FUNCTION "Gest Aut Boxing SX" : VOID
TITLE =Gestione Automatico Boxing SX
AUTHOR : MassimoZ
FAMILY : NovaSrl
VERSION : 0.1

BEGIN
NETWORK
TITLE ======== Automatico Pintaggio Elementi Boxing SX ======



NETWORK
TITLE =Presenza Pezzo su Dosatore in Entrata Boxing SX

      U(    ;
      UN    "SL710";
      U     "SL710B";
      U     "FT502";
      L     S5T#500MS;
      SE    T     86;
      NOP   0;
      NOP   0;
      NOP   0;
      U     T     86;
      )     ;
      L     S5T#700MS;
      SA    T     87;
      NOP   0;
      NOP   0;
      NOP   0;
      U     T     87;
      =     "M90.0";
NETWORK
TITLE =Presenza Pezzo su Prima Zona di Lavoro Boxing SX

      U(    ;
      UN    "SL710";
      U     "SL710B";
      U     "FT504";
      L     S5T#500MS;
      SE    T     88;
      NOP   0;
      NOP   0;
      NOP   0;
      U     T     88;
      )     ;
      L     S5T#300MS;
      SA    T     89;
      NOP   0;
      NOP   0;
      NOP   0;
      U     T     89;
      =     "M90.1";
NETWORK
TITLE =Presenza Pezzo su Seconda Zona di Lavoro Boxing SX

      U(    ;
      UN    "SL710";
      U     "SL710B";
      U     "FT506";
      L     S5T#500MS;
      SE    T     90;
      NOP   0;
      NOP   0;
      NOP   0;
      U     T     90;
      )     ;
      L     S5T#300MS;
      SA    T     91;
      NOP   0;
      NOP   0;
      NOP   0;
      U     T     91;
      =     "M90.2";
NETWORK
TITLE =Presenza Pezzo su Terza Zona di Lavoro Boxing SX

      U(    ;
      UN    "SL710";
      U     "SL710B";
      U     "FT510";
      L     S5T#500MS;
      SE    T     92;
      NOP   0;
      NOP   0;
      NOP   0;
      U     T     92;
      )     ;
      L     S5T#300MS;
      SA    T     93;
      NOP   0;
      NOP   0;
      NOP   0;
      U     T     93;
      =     "M90.3";
NETWORK
TITLE =Com Aut Start Motore Nastro 3
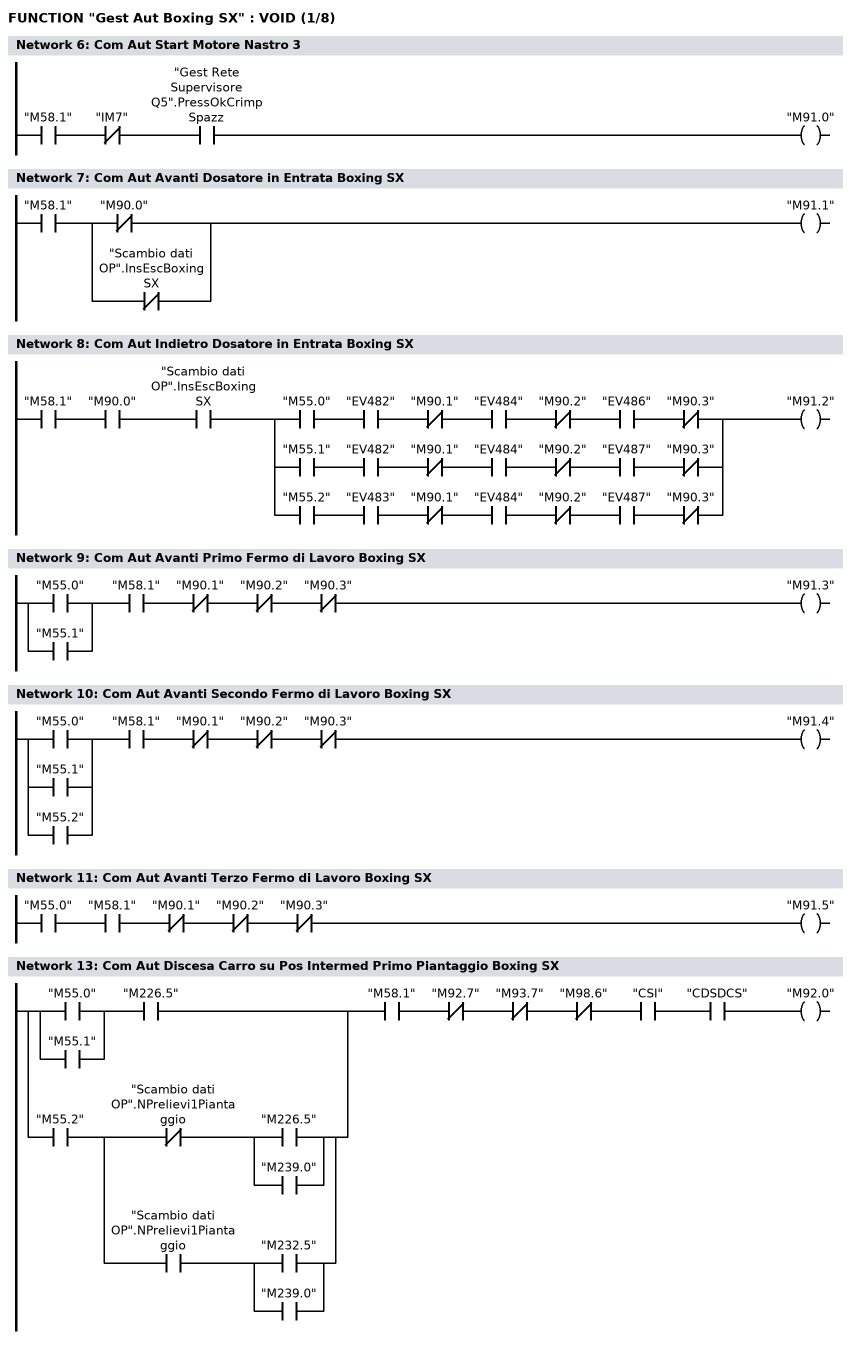
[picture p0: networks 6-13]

      U     "M58.1";
      UN    "IM7";
      U     "Gest Rete Supervisore Q5".PressOkCrimpSpazz;
      =     "M91.0";
NETWORK
TITLE =Com Aut Avanti Dosatore in Entrata Boxing SX

      U     "M58.1";
      U(    ;
      ON    "M90.0";
      ON    "Scambio dati OP".InsEscBoxingSX;
      )     ;
      =     "M91.1";
NETWORK
TITLE =Com Aut Indietro Dosatore in Entrata Boxing SX

      U     "M58.1";
      U     "M90.0";
      U     "Scambio dati OP".InsEscBoxingSX;
      U(    ;
      U     "M55.0";
      U     "EV482";
      UN    "M90.1";
      U     "EV484";
      UN    "M90.2";
      U     "EV486";
      UN    "M90.3";
      O     ;
      U     "M55.1";
      U     "EV482";
      UN    "M90.1";
      U     "EV484";
      UN    "M90.2";
      U     "EV487";
      UN    "M90.3";
      O     ;
      U     "M55.2";
      U     "EV483";
      UN    "M90.1";
      U     "EV484";
      UN    "M90.2";
      U     "EV487";
      UN    "M90.3";
      )     ;
      =     "M91.2";
NETWORK
TITLE =Com Aut Avanti Primo Fermo di Lavoro Boxing SX

      U(    ;
      O     "M55.0";
      O     "M55.1";
      )     ;
      U     "M58.1";
      UN    "M90.1";
      UN    "M90.2";
      UN    "M90.3";
      =     "M91.3";
NETWORK
TITLE =Com Aut Avanti Secondo Fermo di Lavoro Boxing SX

      U(    ;
      O     "M55.0";
      O     "M55.1";
      O     "M55.2";
      )     ;
      U     "M58.1";
      UN    "M90.1";
      UN    "M90.2";
      UN    "M90.3";
      =     "M91.4";
NETWORK
TITLE =Com Aut Avanti Terzo Fermo di Lavoro Boxing SX

      U     "M55.0";
      U     "M58.1";
      UN    "M90.1";
      UN    "M90.2";
      UN    "M90.3";
      =     "M91.5";
NETWORK
TITLE ======= Primo Piantag per Batterie 12V 16V e Batterie in Linea ==



NETWORK
TITLE =Com Aut Discesa Carro su Pos Intermed Primo Piantaggio Boxing SX

      U(    ;
      U(    ;
      O     "M55.0";
      O     "M55.1";
      )     ;
      U     "M226.5";
      O     ;
      U     "M55.2";
      U(    ;
      UN    "Scambio dati OP".NPrelievi1Piantaggio;
      U(    ;
      O     "M226.5";
      O     "M239.0";
      )     ;
      O     ;
      U     "Scambio dati OP".NPrelievi1Piantaggio;
      U(    ;
      O     "M232.5";
      O     "M239.0";
      )     ;
      )     ;
      )     ;
      U     "M58.1";
      UN    "M92.7";
      UN    "M93.7";
      UN    "M98.6";
      U     "CSI";
      U     "CDSDCS";
      =     "M92.0";
NETWORK
TITLE =Com Aut Avanti Carro Primo Piantaggio Boxing SX
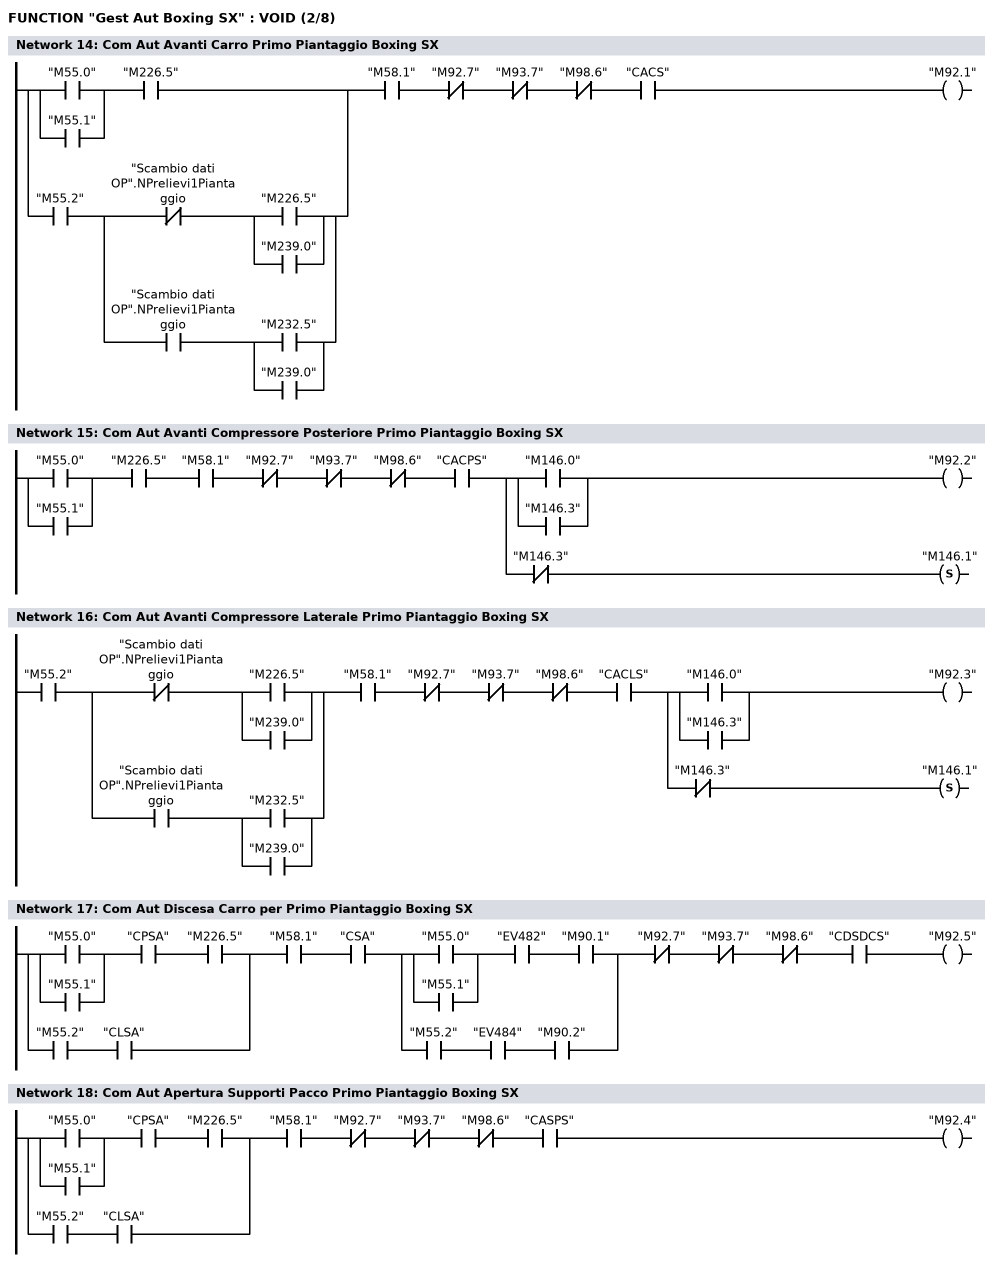
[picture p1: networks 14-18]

      U(    ;
      U(    ;
      O     "M55.0";
      O     "M55.1";
      )     ;
      U     "M226.5";
      O     ;
      U     "M55.2";
      U(    ;
      UN    "Scambio dati OP".NPrelievi1Piantaggio;
      U(    ;
      O     "M226.5";
      O     "M239.0";
      )     ;
      O     ;
      U     "Scambio dati OP".NPrelievi1Piantaggio;
      U(    ;
      O     "M232.5";
      O     "M239.0";
      )     ;
      )     ;
      )     ;
      U     "M58.1";
      UN    "M92.7";
      UN    "M93.7";
      UN    "M98.6";
      U     "CACS";
      =     "M92.1";
NETWORK
TITLE =Com Aut Avanti Compressore Posteriore Primo Piantaggio Boxing SX

      U(    ;
      O     "M55.0";
      O     "M55.1";
      )     ;
      U     "M226.5";
      U     "M58.1";
      UN    "M92.7";
      UN    "M93.7";
      UN    "M98.6";
      U     "CACPS";
      =     L      0.0;
      U     L      0.0;
      U(    ;
      O     "M146.0";
      O     "M146.3";
      )     ;
      =     "M92.2";
      U     L      0.0;
      UN    "M146.3";
      S     "M146.1";
NETWORK
TITLE =Com Aut Avanti Compressore Laterale Primo Piantaggio Boxing SX

      U     "M55.2";
      U(    ;
      UN    "Scambio dati OP".NPrelievi1Piantaggio;
      U(    ;
      O     "M226.5";
      O     "M239.0";
      )     ;
      O     ;
      U     "Scambio dati OP".NPrelievi1Piantaggio;
      U(    ;
      O     "M232.5";
      O     "M239.0";
      )     ;
      )     ;
      U     "M58.1";
      UN    "M92.7";
      UN    "M93.7";
      UN    "M98.6";
      U     "CACLS";
      =     L      0.0;
      U     L      0.0;
      U(    ;
      O     "M146.0";
      O     "M146.3";
      )     ;
      =     "M92.3";
      U     L      0.0;
      UN    "M146.3";
      S     "M146.1";
NETWORK
TITLE =Com Aut Discesa Carro per Primo Piantaggio Boxing SX

      U(    ;
      U(    ;
      O     "M55.0";
      O     "M55.1";
      )     ;
      U     "CPSA";
      U     "M226.5";
      O     ;
      U     "M55.2";
      U     "CLSA";
      )     ;
      U     "M58.1";
      U     "CSA";
      U(    ;
      U(    ;
      O     "M55.0";
      O     "M55.1";
      )     ;
      U     "EV482";
      U     "M90.1";
      O     ;
      U     "M55.2";
      U     "EV484";
      U     "M90.2";
      )     ;
      UN    "M92.7";
      UN    "M93.7";
      UN    "M98.6";
      U     "CDSDCS";
      =     "M92.5";
NETWORK
TITLE =Com Aut Apertura Supporti Pacco Primo Piantaggio Boxing SX

      U(    ;
      U(    ;
      O     "M55.0";
      O     "M55.1";
      )     ;
      U     "CPSA";
      U     "M226.5";
      O     ;
      U     "M55.2";
      U     "CLSA";
      )     ;
      U     "M58.1";
      UN    "M92.7";
      UN    "M93.7";
      UN    "M98.6";
      U     "CASPS";
      =     "M92.4";
NETWORK
TITLE =Com Aut Avanti Blocc Pezzo Zona Lavoro Primo Piantagg Boxing SX
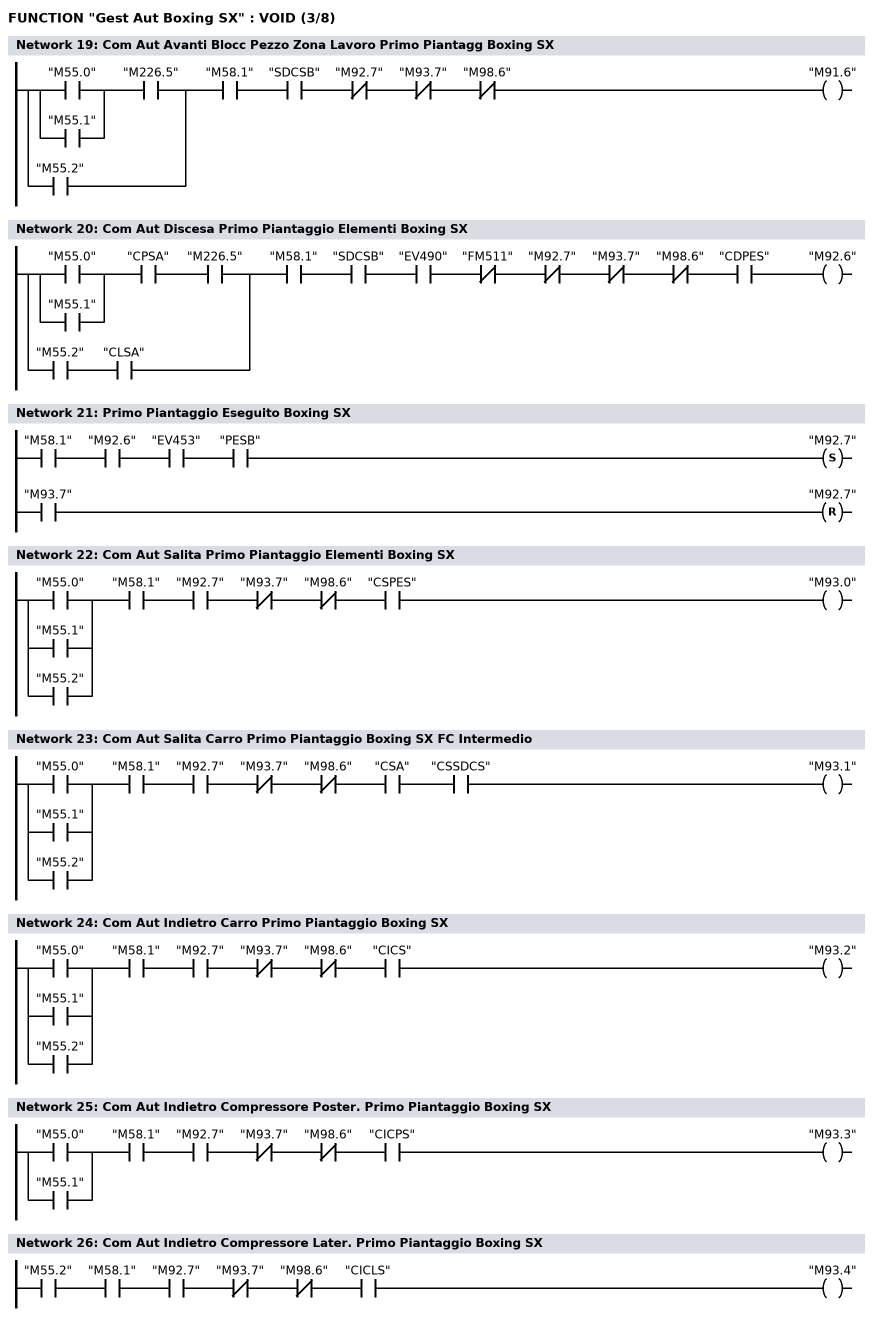
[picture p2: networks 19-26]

      U(    ;
      U(    ;
      O     "M55.0";
      O     "M55.1";
      )     ;
      U     "M226.5";
      O     "M55.2";
      )     ;
      U     "M58.1";
      U     "SDCSB";
      UN    "M92.7";
      UN    "M93.7";
      UN    "M98.6";
      =     "M91.6";
NETWORK
TITLE =Com Aut Discesa Primo Piantaggio Elementi Boxing SX

      U(    ;
      U(    ;
      O     "M55.0";
      O     "M55.1";
      )     ;
      U     "CPSA";
      U     "M226.5";
      O     ;
      U     "M55.2";
      U     "CLSA";
      )     ;
      U     "M58.1";
      U     "SDCSB";
      U     "EV490";
      UN    "FM511";
      UN    "M92.7";
      UN    "M93.7";
      UN    "M98.6";
      U     "CDPES";
      =     "M92.6";
NETWORK
TITLE =Primo Piantaggio Eseguito Boxing SX

      U     "M58.1";
      U     "M92.6";
      U     "EV453";
      U     "PESB";
      S     "M92.7";
      U     "M93.7";
      R     "M92.7";
      NOP   0;
NETWORK
TITLE =Com Aut Salita Primo Piantaggio Elementi Boxing SX

      U(    ;
      O     "M55.0";
      O     "M55.1";
      O     "M55.2";
      )     ;
      U     "M58.1";
      U     "M92.7";
      UN    "M93.7";
      UN    "M98.6";
      U     "CSPES";
      =     "M93.0";
NETWORK
TITLE =Com Aut Salita Carro Primo Piantaggio Boxing SX FC Intermedio

      U(    ;
      O     "M55.0";
      O     "M55.1";
      O     "M55.2";
      )     ;
      U     "M58.1";
      U     "M92.7";
      UN    "M93.7";
      UN    "M98.6";
      U     "CSA";
      U     "CSSDCS";
      =     "M93.1";
NETWORK
TITLE =Com Aut Indietro Carro Primo Piantaggio Boxing SX

      U(    ;
      O     "M55.0";
      O     "M55.1";
      O     "M55.2";
      )     ;
      U     "M58.1";
      U     "M92.7";
      UN    "M93.7";
      UN    "M98.6";
      U     "CICS";
      =     "M93.2";
NETWORK
TITLE =Com Aut Indietro Compressore Poster. Primo Piantaggio Boxing SX

      U(    ;
      O     "M55.0";
      O     "M55.1";
      )     ;
      U     "M58.1";
      U     "M92.7";
      UN    "M93.7";
      UN    "M98.6";
      U     "CICPS";
      =     "M93.3";
NETWORK
TITLE =Com Aut Indietro Compressore Later. Primo Piantaggio Boxing SX

      U     "M55.2";
      U     "M58.1";
      U     "M92.7";
      UN    "M93.7";
      UN    "M98.6";
      U     "CICLS";
      =     "M93.4";
NETWORK
TITLE =Com Aut Chiusura Supporto Pacchi Primo Piantaggio Boxing SX
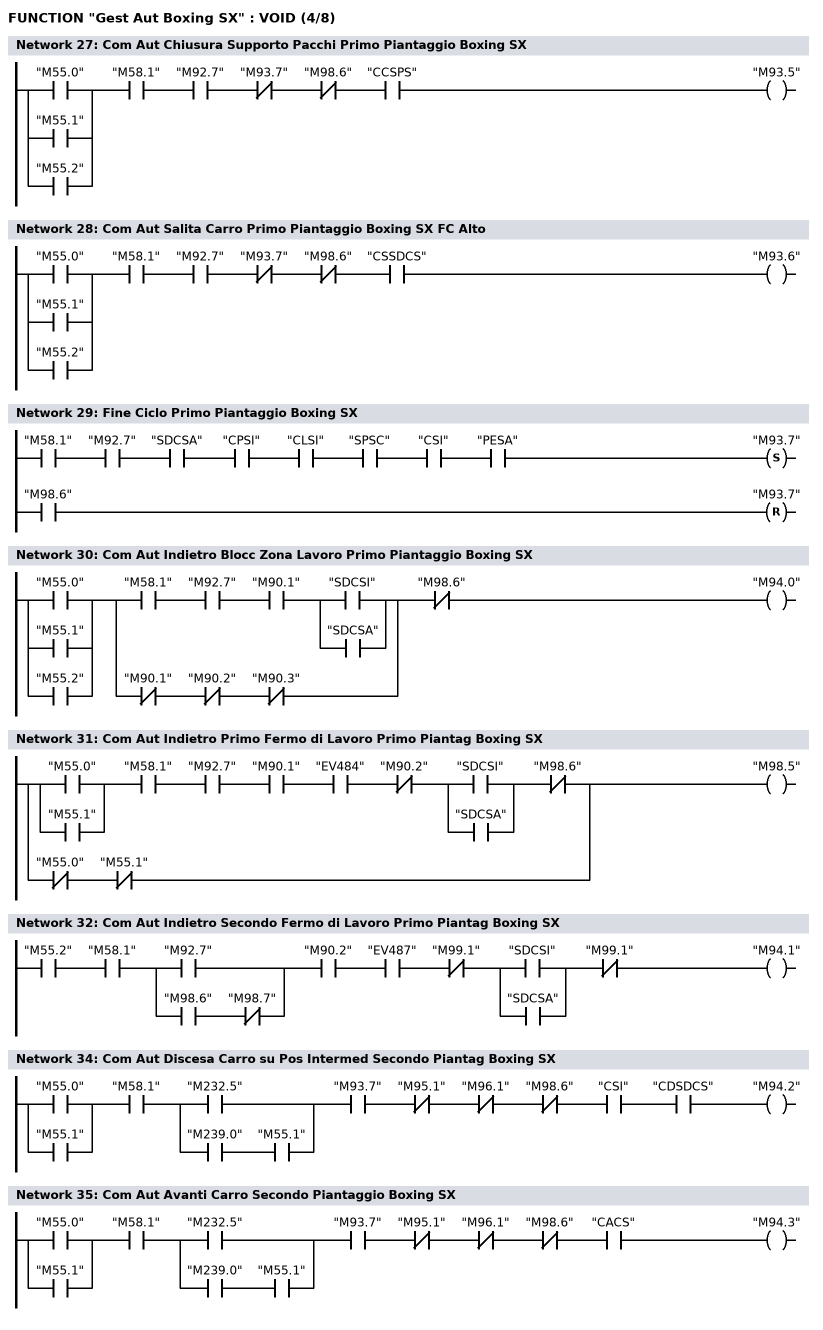
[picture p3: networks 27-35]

      U(    ;
      O     "M55.0";
      O     "M55.1";
      O     "M55.2";
      )     ;
      U     "M58.1";
      U     "M92.7";
      UN    "M93.7";
      UN    "M98.6";
      U     "CCSPS";
      =     "M93.5";
NETWORK
TITLE =Com Aut Salita Carro Primo Piantaggio Boxing SX FC Alto

      U(    ;
      O     "M55.0";
      O     "M55.1";
      O     "M55.2";
      )     ;
      U     "M58.1";
      U     "M92.7";
      UN    "M93.7";
      UN    "M98.6";
      U     "CSSDCS";
      =     "M93.6";
NETWORK
TITLE =Fine Ciclo Primo Piantaggio Boxing SX

      U     "M58.1";
      U     "M92.7";
      U     "SDCSA";
      U     "CPSI";
      U     "CLSI";
      U     "SPSC";
      U     "CSI";
      U     "PESA";
      S     "M93.7";
      U     "M98.6";
      R     "M93.7";
      NOP   0;
NETWORK
TITLE =Com Aut Indietro Blocc Zona Lavoro Primo Piantaggio Boxing SX

      U(    ;
      O     "M55.0";
      O     "M55.1";
      O     "M55.2";
      )     ;
      U(    ;
      U     "M58.1";
      U     "M92.7";
      U     "M90.1";
      U(    ;
      O     "SDCSI";
      O     "SDCSA";
      )     ;
      O     ;
      UN    "M90.1";
      UN    "M90.2";
      UN    "M90.3";
      )     ;
      UN    "M98.6";
      =     "M94.0";
NETWORK
TITLE =Com Aut Indietro Primo Fermo di Lavoro Primo Piantag Boxing SX

      U(    ;
      O     "M55.0";
      O     "M55.1";
      )     ;
      U     "M58.1";
      U     "M92.7";
      U     "M90.1";
      U     "EV484";
      UN    "M90.2";
      U(    ;
      O     "SDCSI";
      O     "SDCSA";
      )     ;
      UN    "M98.6";
      O     ;
      UN    "M55.0";
      UN    "M55.1";
      =     "M98.5";
NETWORK
TITLE =Com Aut Indietro Secondo Fermo di Lavoro Primo Piantag Boxing SX

      U     "M55.2";
      U     "M58.1";
      U(    ;
      O     "M92.7";
      O     ;
      U     "M98.6";
      UN    "M98.7";
      )     ;
      U     "M90.2";
      U     "EV487";
      UN    "M99.1";
      U(    ;
      O     "SDCSI";
      O     "SDCSA";
      )     ;
      UN    "M99.1";
      =     "M94.1";
NETWORK
TITLE ======= Secondo Pinataggio per Batterie 12V 16V =======



NETWORK
TITLE =Com Aut Discesa Carro su Pos Intermed Secondo Piantag Boxing SX

      U(    ;
      O     "M55.0";
      O     "M55.1";
      )     ;
      U     "M58.1";
      U(    ;
      O     "M232.5";
      O     ;
      U     "M239.0";
      U     "M55.1";
      )     ;
      U     "M93.7";
      UN    "M95.1";
      UN    "M96.1";
      UN    "M98.6";
      U     "CSI";
      U     "CDSDCS";
      =     "M94.2";
NETWORK
TITLE =Com Aut Avanti Carro Secondo Piantaggio Boxing SX

      U(    ;
      O     "M55.0";
      O     "M55.1";
      )     ;
      U     "M58.1";
      U(    ;
      O     "M232.5";
      O     ;
      U     "M239.0";
      U     "M55.1";
      )     ;
      U     "M93.7";
      UN    "M95.1";
      UN    "M96.1";
      UN    "M98.6";
      U     "CACS";
      =     "M94.3";
NETWORK
TITLE =Com Aut Avanti Compressore Posteriore Secondo Piantag Boxing SX
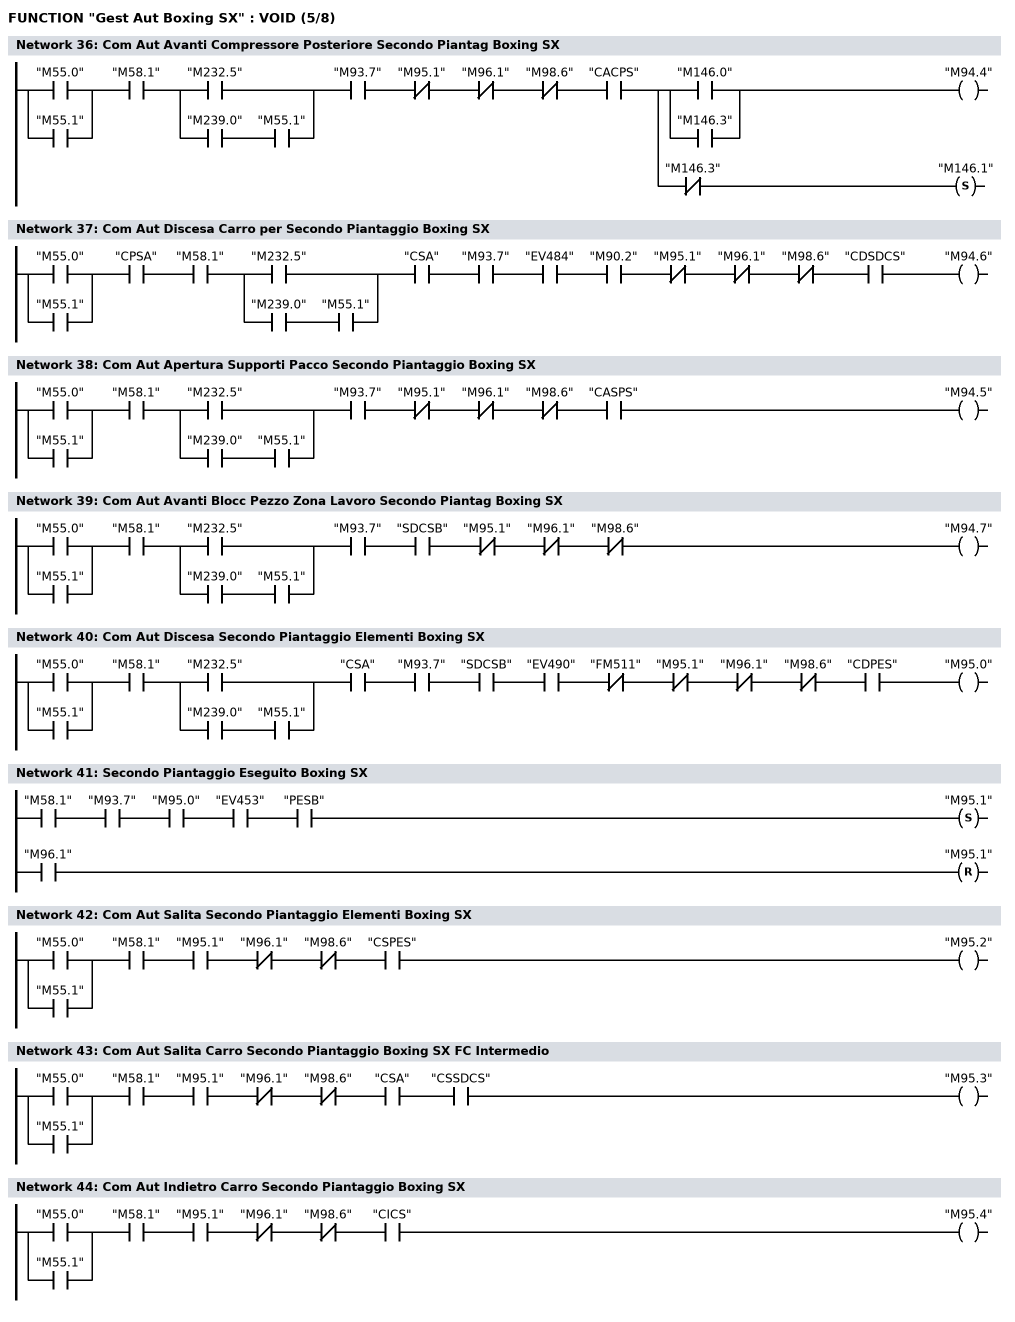
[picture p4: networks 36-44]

      U(    ;
      O     "M55.0";
      O     "M55.1";
      )     ;
      U     "M58.1";
      U(    ;
      O     "M232.5";
      O     ;
      U     "M239.0";
      U     "M55.1";
      )     ;
      U     "M93.7";
      UN    "M95.1";
      UN    "M96.1";
      UN    "M98.6";
      U     "CACPS";
      =     L      0.0;
      U     L      0.0;
      U(    ;
      O     "M146.0";
      O     "M146.3";
      )     ;
      =     "M94.4";
      U     L      0.0;
      UN    "M146.3";
      S     "M146.1";
NETWORK
TITLE =Com Aut Discesa Carro per Secondo Piantaggio Boxing SX

      U(    ;
      O     "M55.0";
      O     "M55.1";
      )     ;
      U     "CPSA";
      U     "M58.1";
      U(    ;
      O     "M232.5";
      O     ;
      U     "M239.0";
      U     "M55.1";
      )     ;
      U     "CSA";
      U     "M93.7";
      U     "EV484";
      U     "M90.2";
      UN    "M95.1";
      UN    "M96.1";
      UN    "M98.6";
      U     "CDSDCS";
      =     "M94.6";
NETWORK
TITLE =Com Aut Apertura Supporti Pacco Secondo Piantaggio Boxing SX

      U(    ;
      O     "M55.0";
      O     "M55.1";
      )     ;
      U     "M58.1";
      U(    ;
      O     "M232.5";
      O     ;
      U     "M239.0";
      U     "M55.1";
      )     ;
      U     "M93.7";
      UN    "M95.1";
      UN    "M96.1";
      UN    "M98.6";
      U     "CASPS";
      =     "M94.5";
NETWORK
TITLE =Com Aut Avanti Blocc Pezzo Zona Lavoro Secondo Piantag Boxing SX

      U(    ;
      O     "M55.0";
      O     "M55.1";
      )     ;
      U     "M58.1";
      U(    ;
      O     "M232.5";
      O     ;
      U     "M239.0";
      U     "M55.1";
      )     ;
      U     "M93.7";
      U     "SDCSB";
      UN    "M95.1";
      UN    "M96.1";
      UN    "M98.6";
      =     "M94.7";
NETWORK
TITLE =Com Aut Discesa Secondo Piantaggio Elementi Boxing SX

      U(    ;
      O     "M55.0";
      O     "M55.1";
      )     ;
      U     "M58.1";
      U(    ;
      O     "M232.5";
      O     ;
      U     "M239.0";
      U     "M55.1";
      )     ;
      U     "CSA";
      U     "M93.7";
      U     "SDCSB";
      U     "EV490";
      UN    "FM511";
      UN    "M95.1";
      UN    "M96.1";
      UN    "M98.6";
      U     "CDPES";
      =     "M95.0";
NETWORK
TITLE =Secondo Piantaggio Eseguito Boxing SX

      U     "M58.1";
      U     "M93.7";
      U     "M95.0";
      U     "EV453";
      U     "PESB";
      S     "M95.1";
      U     "M96.1";
      R     "M95.1";
      NOP   0;
NETWORK
TITLE =Com Aut Salita Secondo Piantaggio Elementi Boxing SX

      U(    ;
      O     "M55.0";
      O     "M55.1";
      )     ;
      U     "M58.1";
      U     "M95.1";
      UN    "M96.1";
      UN    "M98.6";
      U     "CSPES";
      =     "M95.2";
NETWORK
TITLE =Com Aut Salita Carro Secondo Piantaggio Boxing SX FC Intermedio

      U(    ;
      O     "M55.0";
      O     "M55.1";
      )     ;
      U     "M58.1";
      U     "M95.1";
      UN    "M96.1";
      UN    "M98.6";
      U     "CSA";
      U     "CSSDCS";
      =     "M95.3";
NETWORK
TITLE =Com Aut Indietro Carro Secondo Piantaggio Boxing SX

      U(    ;
      O     "M55.0";
      O     "M55.1";
      )     ;
      U     "M58.1";
      U     "M95.1";
      UN    "M96.1";
      UN    "M98.6";
      U     "CICS";
      =     "M95.4";
NETWORK
TITLE =Com Aut Indietro Compressore Poster. Secondo Piantag Boxing SX
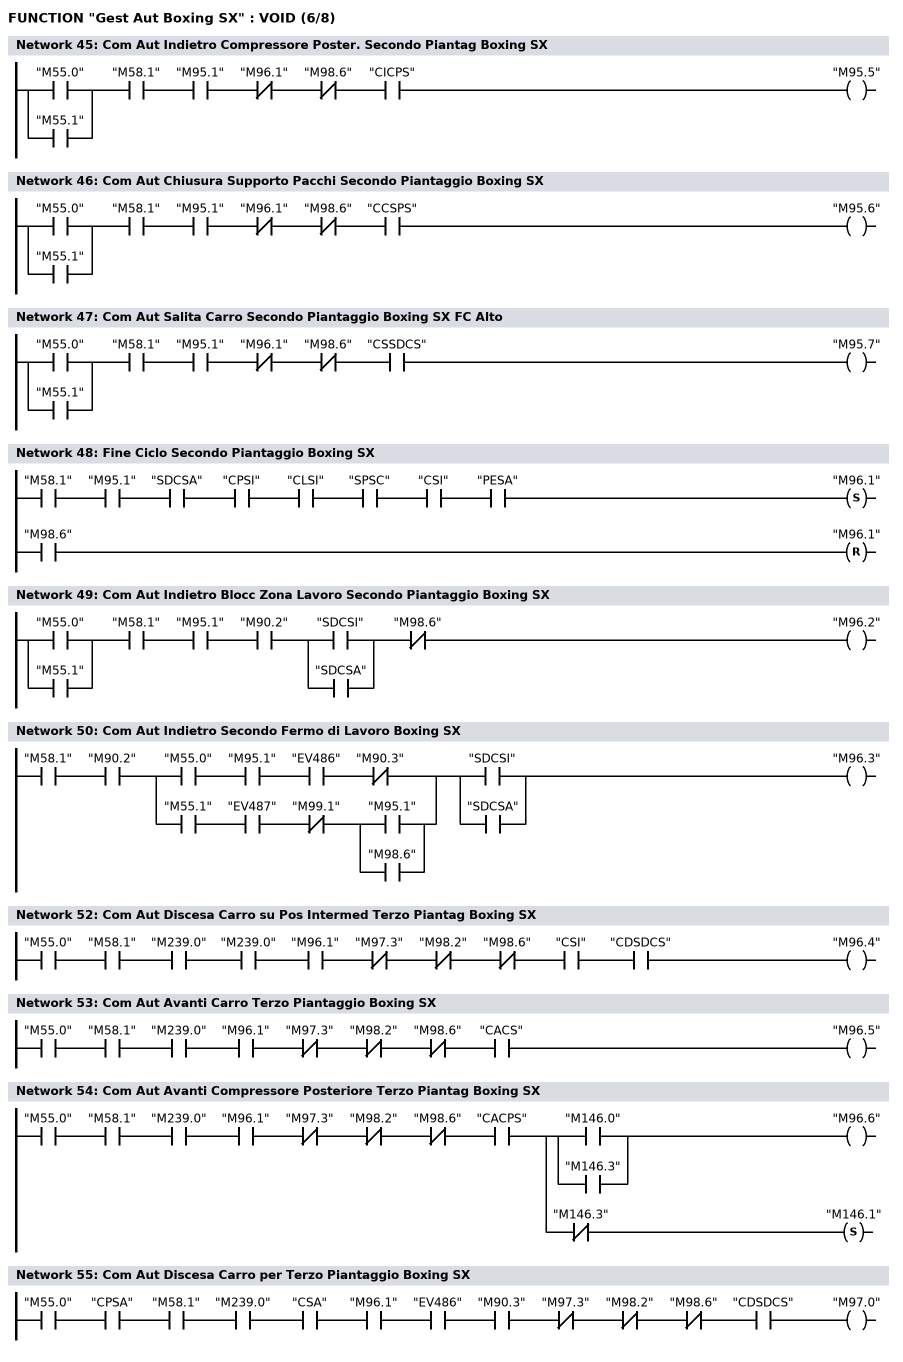
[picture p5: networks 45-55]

      U(    ;
      O     "M55.0";
      O     "M55.1";
      )     ;
      U     "M58.1";
      U     "M95.1";
      UN    "M96.1";
      UN    "M98.6";
      U     "CICPS";
      =     "M95.5";
NETWORK
TITLE =Com Aut Chiusura Supporto Pacchi Secondo Piantaggio Boxing SX

      U(    ;
      O     "M55.0";
      O     "M55.1";
      )     ;
      U     "M58.1";
      U     "M95.1";
      UN    "M96.1";
      UN    "M98.6";
      U     "CCSPS";
      =     "M95.6";
NETWORK
TITLE =Com Aut Salita Carro Secondo Piantaggio Boxing SX FC Alto

      U(    ;
      O     "M55.0";
      O     "M55.1";
      )     ;
      U     "M58.1";
      U     "M95.1";
      UN    "M96.1";
      UN    "M98.6";
      U     "CSSDCS";
      =     "M95.7";
NETWORK
TITLE =Fine Ciclo Secondo Piantaggio Boxing SX

      U     "M58.1";
      U     "M95.1";
      U     "SDCSA";
      U     "CPSI";
      U     "CLSI";
      U     "SPSC";
      U     "CSI";
      U     "PESA";
      S     "M96.1";
      U     "M98.6";
      R     "M96.1";
      NOP   0;
NETWORK
TITLE =Com Aut Indietro Blocc Zona Lavoro Secondo Piantaggio Boxing SX

      U(    ;
      O     "M55.0";
      O     "M55.1";
      )     ;
      U     "M58.1";
      U     "M95.1";
      U     "M90.2";
      U(    ;
      O     "SDCSI";
      O     "SDCSA";
      )     ;
      UN    "M98.6";
      =     "M96.2";
NETWORK
TITLE =Com Aut Indietro Secondo Fermo di Lavoro Boxing SX

      U     "M58.1";
      U     "M90.2";
      U(    ;
      U     "M55.0";
      U     "M95.1";
      U     "EV486";
      UN    "M90.3";
      O     ;
      U     "M55.1";
      U     "EV487";
      UN    "M99.1";
      U(    ;
      O     "M95.1";
      O     "M98.6";
      )     ;
      )     ;
      U(    ;
      O     "SDCSI";
      O     "SDCSA";
      )     ;
      =     "M96.3";
NETWORK
TITLE ======= Terzo Pinataggio per Batterie 12V  =======



NETWORK
TITLE =Com Aut Discesa Carro su Pos Intermed Terzo Piantag Boxing SX

      U     "M55.0";
      U     "M58.1";
      U     "M239.0";
      U     "M239.0";
      U     "M96.1";
      UN    "M97.3";
      UN    "M98.2";
      UN    "M98.6";
      U     "CSI";
      U     "CDSDCS";
      =     "M96.4";
NETWORK
TITLE =Com Aut Avanti Carro Terzo Piantaggio Boxing SX

      U     "M55.0";
      U     "M58.1";
      U     "M239.0";
      U     "M96.1";
      UN    "M97.3";
      UN    "M98.2";
      UN    "M98.6";
      U     "CACS";
      =     "M96.5";
NETWORK
TITLE =Com Aut Avanti Compressore Posteriore Terzo Piantag Boxing SX

      U     "M55.0";
      U     "M58.1";
      U     "M239.0";
      U     "M96.1";
      UN    "M97.3";
      UN    "M98.2";
      UN    "M98.6";
      U     "CACPS";
      =     L      0.0;
      U     L      0.0;
      U(    ;
      O     "M146.0";
      O     "M146.3";
      )     ;
      =     "M96.6";
      U     L      0.0;
      UN    "M146.3";
      S     "M146.1";
NETWORK
TITLE =Com Aut Discesa Carro per Terzo Piantaggio Boxing SX

      U     "M55.0";
      U     "CPSA";
      U     "M58.1";
      U     "M239.0";
      U     "CSA";
      U     "M96.1";
      U     "EV486";
      U     "M90.3";
      UN    "M97.3";
      UN    "M98.2";
      UN    "M98.6";
      U     "CDSDCS";
      =     "M97.0";
NETWORK
TITLE =Com Aut Apertura Supporti Pacco Terzo Piantaggio Boxing SX
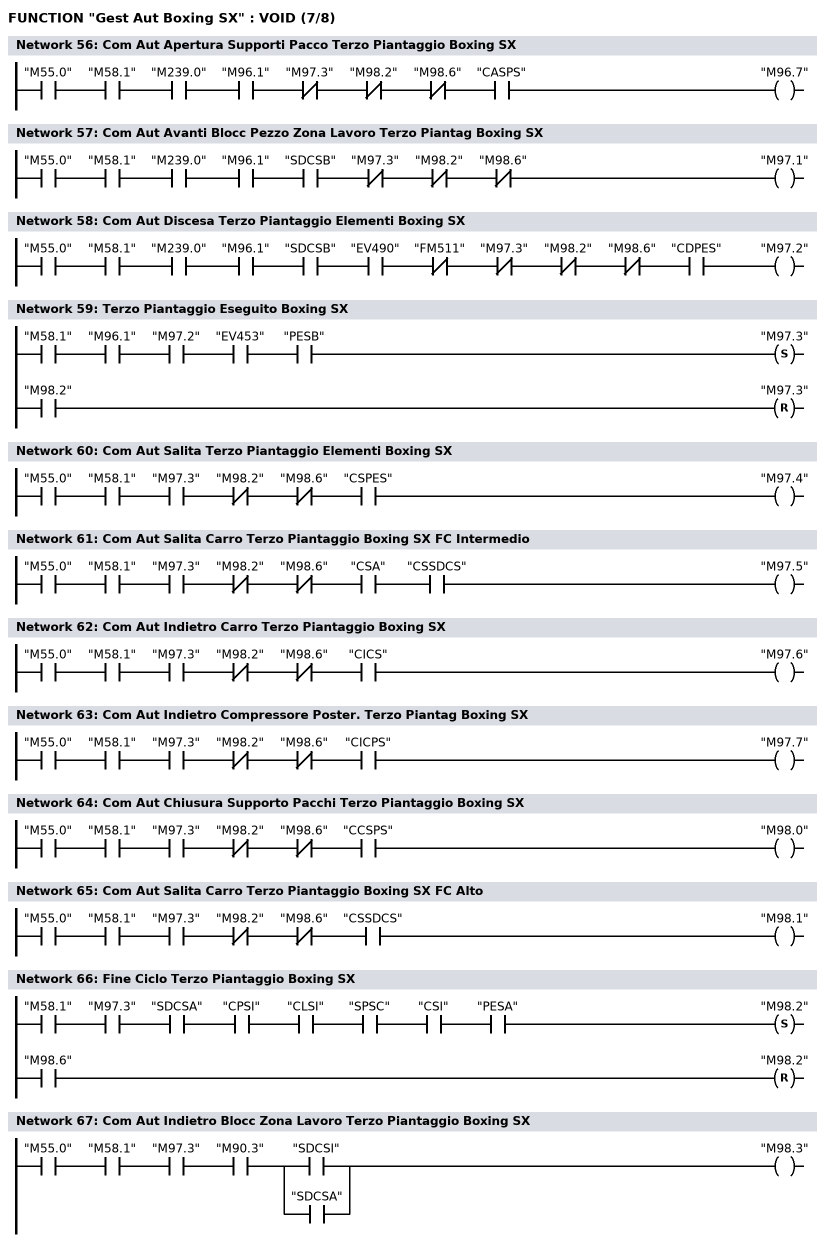
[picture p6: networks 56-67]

      U     "M55.0";
      U     "M58.1";
      U     "M239.0";
      U     "M96.1";
      UN    "M97.3";
      UN    "M98.2";
      UN    "M98.6";
      U     "CASPS";
      =     "M96.7";
NETWORK
TITLE =Com Aut Avanti Blocc Pezzo Zona Lavoro Terzo Piantag Boxing SX

      U     "M55.0";
      U     "M58.1";
      U     "M239.0";
      U     "M96.1";
      U     "SDCSB";
      UN    "M97.3";
      UN    "M98.2";
      UN    "M98.6";
      =     "M97.1";
NETWORK
TITLE =Com Aut Discesa Terzo Piantaggio Elementi Boxing SX

      U     "M55.0";
      U     "M58.1";
      U     "M239.0";
      U     "M96.1";
      U     "SDCSB";
      U     "EV490";
      UN    "FM511";
      UN    "M97.3";
      UN    "M98.2";
      UN    "M98.6";
      U     "CDPES";
      =     "M97.2";
NETWORK
TITLE =Terzo Piantaggio Eseguito Boxing SX

      U     "M58.1";
      U     "M96.1";
      U     "M97.2";
      U     "EV453";
      U     "PESB";
      S     "M97.3";
      U     "M98.2";
      R     "M97.3";
      NOP   0;
NETWORK
TITLE =Com Aut Salita Terzo Piantaggio Elementi Boxing SX

      U     "M55.0";
      U     "M58.1";
      U     "M97.3";
      UN    "M98.2";
      UN    "M98.6";
      U     "CSPES";
      =     "M97.4";
NETWORK
TITLE =Com Aut Salita Carro Terzo Piantaggio Boxing SX FC Intermedio

      U     "M55.0";
      U     "M58.1";
      U     "M97.3";
      UN    "M98.2";
      UN    "M98.6";
      U     "CSA";
      U     "CSSDCS";
      =     "M97.5";
NETWORK
TITLE =Com Aut Indietro Carro Terzo Piantaggio Boxing SX

      U     "M55.0";
      U     "M58.1";
      U     "M97.3";
      UN    "M98.2";
      UN    "M98.6";
      U     "CICS";
      =     "M97.6";
NETWORK
TITLE =Com Aut Indietro Compressore Poster. Terzo Piantag Boxing SX

      U     "M55.0";
      U     "M58.1";
      U     "M97.3";
      UN    "M98.2";
      UN    "M98.6";
      U     "CICPS";
      =     "M97.7";
NETWORK
TITLE =Com Aut Chiusura Supporto Pacchi Terzo Piantaggio Boxing SX

      U     "M55.0";
      U     "M58.1";
      U     "M97.3";
      UN    "M98.2";
      UN    "M98.6";
      U     "CCSPS";
      =     "M98.0";
NETWORK
TITLE =Com Aut Salita Carro Terzo Piantaggio Boxing SX FC Alto

      U     "M55.0";
      U     "M58.1";
      U     "M97.3";
      UN    "M98.2";
      UN    "M98.6";
      U     "CSSDCS";
      =     "M98.1";
NETWORK
TITLE =Fine Ciclo Terzo Piantaggio Boxing SX

      U     "M58.1";
      U     "M97.3";
      U     "SDCSA";
      U     "CPSI";
      U     "CLSI";
      U     "SPSC";
      U     "CSI";
      U     "PESA";
      S     "M98.2";
      U     "M98.6";
      R     "M98.2";
      NOP   0;
NETWORK
TITLE =Com Aut Indietro Blocc Zona Lavoro Terzo Piantaggio Boxing SX

      U     "M55.0";
      U     "M58.1";
      U     "M97.3";
      U     "M90.3";
      U(    ;
      O     "SDCSI";
      O     "SDCSA";
      )     ;
      =     "M98.3";
NETWORK
TITLE =Com Aut Indietro Terzo Fermo di Lavoro Boxing SX
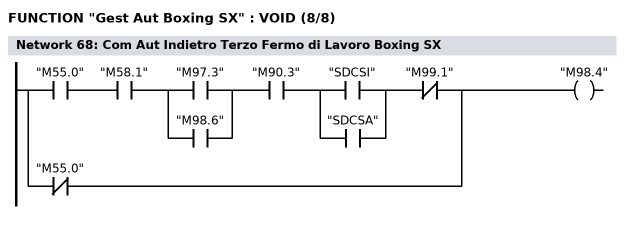
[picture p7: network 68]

      U     "M55.0";
      U     "M58.1";
      U(    ;
      O     "M97.3";
      O     "M98.6";
      )     ;
      U     "M90.3";
      U(    ;
      O     "SDCSI";
      O     "SDCSA";
      )     ;
      UN    "M99.1";
      ON    "M55.0";
      =     "M98.4";
NETWORK
TITLE =Presenza Pezzo su Fermo in Uscita Zona di Lavoro Boxing SX

      U(    ;
      UN    "SL710";
      U     "SL710B";
      U     "FT515";
      L     S5T#2S;
      SE    T     96;
      NOP   0;
      NOP   0;
      NOP   0;
      U     T     96;
      )     ;
      L     S5T#1S;
      SA    T     97;
      NOP   0;
      NOP   0;
      NOP   0;
      U     T     97;
      =     "M99.1";
NETWORK
TITLE =Com Aut Avanti Fermo in Uscita Zona di Lavoro Boxing SX
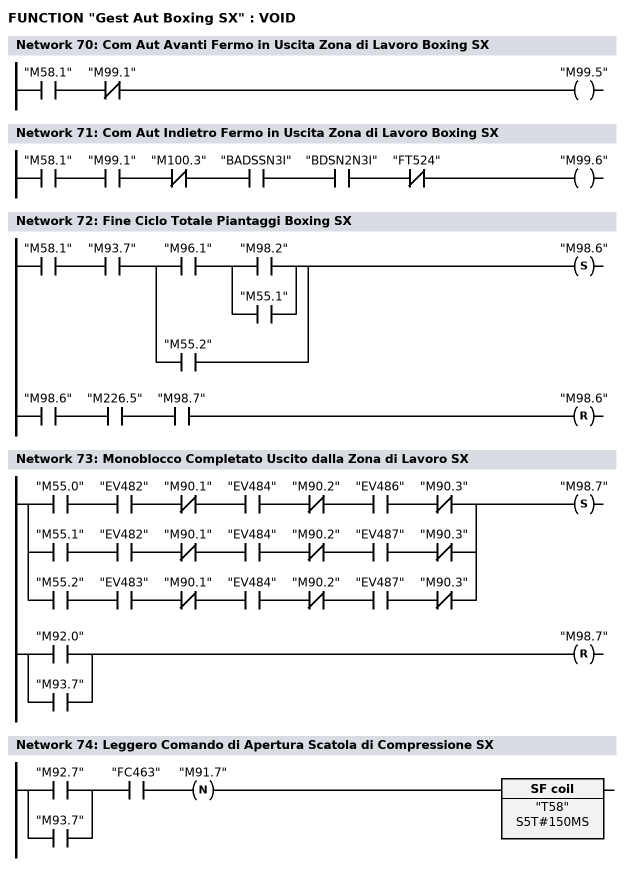
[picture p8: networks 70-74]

      U     "M58.1";
      UN    "M99.1";
      =     "M99.5";
NETWORK
TITLE =Com Aut Indietro Fermo in Uscita Zona di Lavoro Boxing SX

      U     "M58.1";
      U     "M99.1";
      UN    "M100.3";
      U     "BADSSN3I";
      U     "BDSN2N3I";
      UN    "FT524";
      =     "M99.6";
NETWORK
TITLE =Fine Ciclo Totale Piantaggi Boxing SX

      U     "M58.1";
      U     "M93.7";
      U(    ;
      U     "M96.1";
      U(    ;
      O     "M98.2";
      O     "M55.1";
      )     ;
      O     "M55.2";
      )     ;
      S     "M98.6";
      U     "M98.6";
      U     "M226.5";
      U     "M98.7";
      R     "M98.6";
      NOP   0;
NETWORK
TITLE =Monoblocco Completato Uscito dalla Zona di Lavoro SX

      U(    ;
      U     "M55.0";
      U     "EV482";
      UN    "M90.1";
      U     "EV484";
      UN    "M90.2";
      U     "EV486";
      UN    "M90.3";
      O     ;
      U     "M55.1";
      U     "EV482";
      UN    "M90.1";
      U     "EV484";
      UN    "M90.2";
      U     "EV487";
      UN    "M90.3";
      O     ;
      U     "M55.2";
      U     "EV483";
      UN    "M90.1";
      U     "EV484";
      UN    "M90.2";
      U     "EV487";
      UN    "M90.3";
      )     ;
      S     "M98.7";
      U(    ;
      O     "M92.0";
      O     "M93.7";
      )     ;
      R     "M98.7";
      NOP   0;
NETWORK
TITLE =Leggero Comando di Apertura Scatola di Compressione SX

      U(    ;
      O     "M92.7";
      O     "M93.7";
      )     ;
      U     "FC463";
      FN    "M91.7";
      L     S5T#150MS;
      SA    "T58";
NETWORK
TITLE =Numero Cicli Allineatore Guppi Boxing SX

      U(    ;
      U     "M146.1";
      U     "A       5.4";
      UN    "E       5.2";
      =     L      0.0;
      BLD   103;
      U     "M58.1";
      SPBNB _001;
      CALL "TON" , "TON_DB13" (
           IN                       := L      0.0,
           PT                       := T#500MS,
           Q                        := "M146.2");

_001: U     BIE;
      )     ;
      U     "M146.2";
      ZV    "Z5";
NETWORK
TITLE =Comando Allineatori Boxing SX
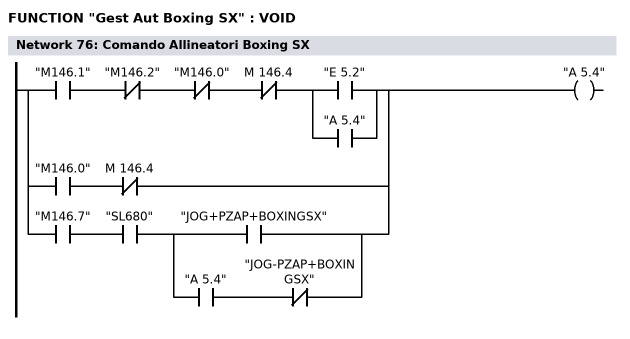
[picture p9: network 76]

      U     "M146.1";
      UN    "M146.2";
      UN    "M146.0";
      UN    M    146.4;
      U(    ;
      O     "E       5.2";
      O     "A       5.4";
      )     ;
      O     ;
      U     "M146.0";
      UN    M    146.4;
      O     ;
      U     "M146.7";
      U     "SL680";
      U(    ;
      O     "JOG+PZAP+BOXINGSX";
      O     ;
      U     "A       5.4";
      UN    "JOG-PZAP+BOXINGSX";
      )     ;
      =     "A       5.4";
NETWORK
TITLE =Fine Ciclo Allineatore Guppi Boxing SX

      L     "Z5";
      L     "Dati".Num_Colpi_All_Gruppi_SX;
      >=I   ;
//      U     E      5.2
      S     "M146.0";
      R     "M146.1";

      U     "M146.0";
      O     "SL710";
      ON    "M58.1";
      O     "M146.3";
      SPBN  M001;
      R     "Z5";
M001: NOP   0;
NETWORK
TITLE =Reset Fine Ciclo Allineatore Guppi Boxing SX
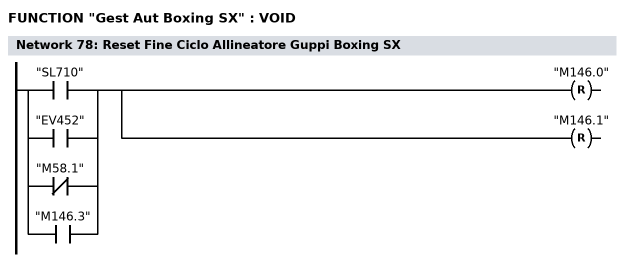
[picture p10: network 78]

      O     "SL710";
      O     "EV452";
      ON    "M58.1";



      O     "M146.3";
      R     "M146.0";
      R     "M146.1";
END_FUNCTION

